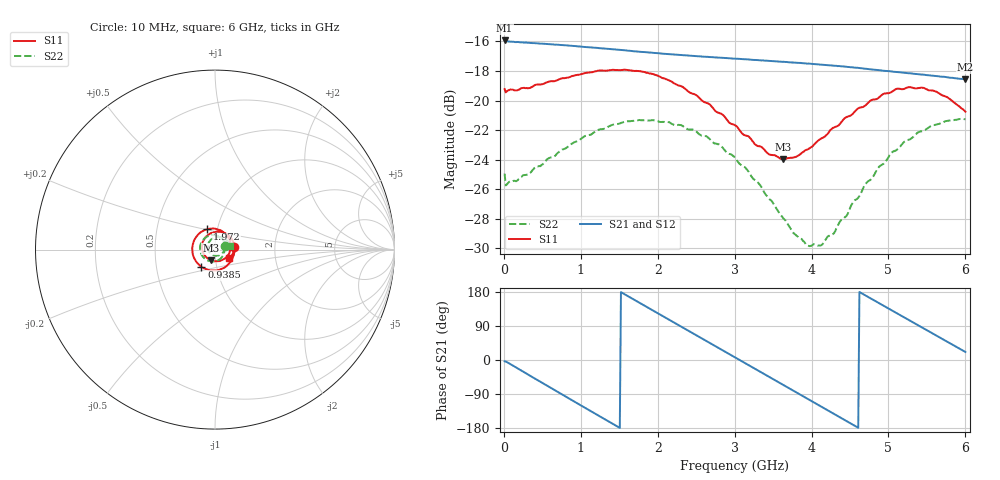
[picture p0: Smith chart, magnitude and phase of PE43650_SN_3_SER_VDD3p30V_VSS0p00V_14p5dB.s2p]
!Keysight Technologies,N5245B,MY57181451,A.13.50.07
!Date: Tuesday, May 07, 2019 08:00:14
!Correction: S11(Full 2 Port(1,2))
!S21(Full 2 Port(1,2))
!S12(Full 2 Port(1,2))
!S22(Full 2 Port(1,2))
!S2P File: Measurements: S11, S21, S12, S22:
# Hz S  dB  R 50
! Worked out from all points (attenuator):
!   401 points, 10 MHz to 6 GHz, reference 50 ohm
!   highest |S21| = -15.93 dB at 10 MHz (marker M1); lowest = -18.6 dB at 6 GHz (marker M2)
!   lowest |S11| = -24.0 dB at 3.634 GHz (marker M3), VSWR 1.14, Z = 47.4 - j5.58 ohm
!   |S11| at or under -10 dB: start of sweep to end of sweep
!   |S22| runs from -29.9 to -21.2 dB; largest |S21 - S12| = 0.0015
!   S11 on the Smith chart (normalised r, x): 10 MHz: 1.24, +0.03; 938.5 MHz: 0.85, -0.16; 1.972 GHz: 0.89, +0.20; 6 GHz: 1.16, -0.12
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1e7  -19.22 7.0  -15.93 -3.5  -16.00 -3.4  -24.94 20.4
1.44775e8  -19.31 -20.9  -16.04 -18.0  -16.07 -18.0  -25.44 -19.6
4.74225e8  -18.91 -67.6  -16.14 -57.4  -16.19 -57.3  -24.44 -66.8
7.13825e8  -18.57 -99.6  -16.23 -85.8  -16.28 -85.8  -23.49 -97.7
9.3845e8  -18.27 -128.1  -16.31 -112.4  -16.37 -112.3  -22.78 -123.6
1.013325e9  -18.21 -137.6  -16.36 -121.2  -16.40 -121.2  -22.54 -132.2
1.252925e9  -17.97 -166.0  -16.45 -149.4  -16.51 -149.3  -21.95 -157.5
1.492525e9  -17.94 166.0  -16.56 -177.4  -16.62 -177.4  -21.57 178.1
1.971725e9  -18.26 112.1  -16.78 126.8  -16.83 126.8  -21.34 131.7
2.01665e9  -18.35 107.0  -16.80 121.5  -16.86 121.5  -21.43 127.4
2.4659e9  -19.55 55.1  -16.98 69.5  -17.04 69.6  -21.99 84.1
2.750425e9  -20.71 21.1  -17.08 36.6  -17.13 36.6  -22.91 56.0
3.005e9  -21.67 -13.0  -17.16 7.1  -17.22 7.2  -23.86 29.9
3.3045e9  -23.08 -57.4  -17.26 -27.6  -17.32 -27.5  -25.55 -5.1
3.63395e9  -23.98 -112.0  -17.37 -65.8  -17.42 -65.8  -27.97 -49.5
3.7837e9  -23.83 -137.7  -17.43 -83.2  -17.48 -83.2  -29.04 -73.8
4.008325e9  -23.11 -174.1  -17.52 -109.3  -17.56 -109.2  -29.79 -116.0
4.277875e9  -21.85 147.4  -17.63 -140.6  -17.68 -140.5  -29.04 -165.9
4.517475e9  -20.98 116.1  -17.74 -168.4  -17.80 -168.2  -27.07 155.5
5.01165e9  -19.48 60.9  -18.01 134.6  -18.06 134.7  -23.72 97.8
5.475875e9  -19.19 14.9  -18.26 81.2  -18.31 81.3  -22.00 54.8
6e9  -20.75 -32.6  -18.56 21.2  -18.61 21.3  -21.26 12.5
